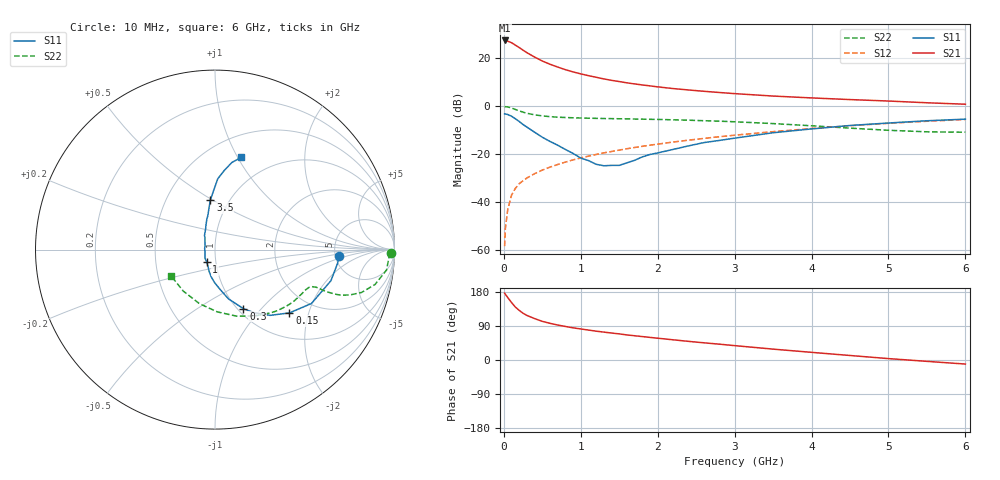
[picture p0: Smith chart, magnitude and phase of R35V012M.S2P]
! SIEMENS Small Signal Semiconductors
! BFR181
! Si NPN RF Bipolar Junction Transistor in SOT23
! VCE = 5 V  IC = 12 mA
! Common Emitter S-Parameters:  May  1996
# GHz  S  MA  R  50
!  f  S11  S21  S12  S22
! GHz  MAG  ANG  MAG  ANG  MAG  ANG  MAG  ANG
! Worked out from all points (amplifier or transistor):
!   36 points, 10 MHz to 6 GHz, reference 50 ohm
!   highest |S21| = 27.4 dB at 10 MHz (marker M1)
!   |S21| within 3 dB of that: start of sweep to 201.7 MHz
!   unconditionally stable (mu >= 1): 748.3 MHz to 2.609 GHz
!   at 250 MHz: K = 0.65, MSG = 27.2 dB, |S12| = -31.1 dB
!   at 1.4 GHz: K = 1.06, MAG = 13.4 dB, |S12| = -18.9 dB
!   at 6 GHz: K = 0.85, MSG = 3.2 dB, |S12| = -5.6 dB
!   S11 on the Smith chart (normalised r, x): 10 MHz: 5.35, -0.71; 150 MHz: 1.51, -1.51; 300 MHz: 1.06, -0.81; 1 GHz: 0.90, -0.12; 3.5 GHz: 0.82, +0.49; 6 GHz: 0.72, +1.04
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0.01  0.6897 -2.9  23.4 176.3  0.0012 81.9  0.9815 -1.2
0.02  0.688 -6.1  23.05 173.3  0.0028 90.0  0.97 -2.7
0.05  0.6688 -15.0  22.61 165.0  0.0069 82.5  0.9625 -6.8
0.1  0.6156 -29.2  21.01 151.6  0.0139 79.0  0.9126 -12.3
0.15  0.5443 -40.4  18.69 139.6  0.0193 72.9  0.8508 -16.3
0.2  0.4776 -50.1  16.64 130.9  0.0241 71.4  0.795 -18.5
0.25  0.4129 -58.3  14.65 123.3  0.0278 69.9  0.7474 -19.9
0.3  0.3651 -64.3  13.01 117.6  0.0317 69.6  0.7085 -20.4
0.4  0.2854 -74.6  10.54 109.3  0.039 69.5  0.6577 -20.7
0.5  0.2244 -82.6  8.713 102.0  0.0463 70.2  0.6257 -20.5
0.6  0.1832 -90.9  7.472 96.8  0.0534 70.9  0.6025 -20.4
0.7  0.1529 -98.0  6.525 92.3  0.0605 71.0  0.5881 -20.7
0.8  0.1247 -105.5  5.757 88.5  0.068 70.9  0.5783 -20.9
1  0.0826 -124.9  4.701 81.9  0.0828 71.1  0.5644 -21.9
1.1  0.0731 -140.0  4.32 79.0  0.0905 71.1  0.5594 -22.7
1.3  0.057 -168.7  3.691 73.6  0.106 70.5  0.5513 -24.3
1.6  0.0656 147.6  3.057 66.2  0.1294 69.3  0.5416 -27.4
2.2  0.125 114.8  2.323 53.3  0.1781 65.9  0.5183 -35.2
3.5  0.2784 95.3  1.621 28.7  0.293 55.0  0.4322 -58.8
4.5  0.3944 87.8  1.369 11.9  0.3902 44.1  0.347 -88.0
5.5  0.4948 79.0  1.174 -3.6  0.4834 31.3  0.291 -127.3
6  0.5345 74.1  1.095 -10.7  0.5263 24.2  0.2853 -149.3
